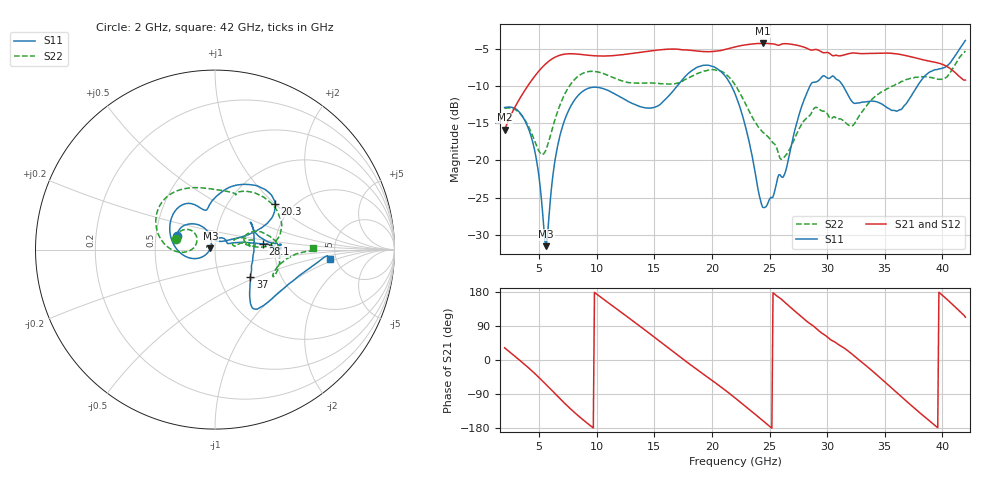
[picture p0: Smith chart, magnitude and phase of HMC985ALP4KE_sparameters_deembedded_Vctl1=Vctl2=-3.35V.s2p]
!s2p File: Measurements: S11, S21, S12, S22
# GHz S dB R 50.0
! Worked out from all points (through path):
!   401 points, 2 GHz to 42 GHz, reference 50 ohm
!   highest |S21| = -4.25 dB at 24.4 GHz (marker M1); lowest = -15.9 dB at 2 GHz (marker M2)
!   lowest |S11| = -31.5 dB at 5.6 GHz (marker M3), VSWR 1.05, Z = 47.5 + j0.726 ohm
!   |S11| at or under -10 dB: start of sweep to 16.97 GHz; 21.7 GHz to 28.5 GHz (6.799 GHz wide, 27.1 % of centre); 31.39 GHz to 37.83 GHz (6.435 GHz wide, 18.6 % of centre)
!   |S22| runs from -19.8 to -5.3 dB; largest |S21 - S12| = 0.00072
!   S11 on the Smith chart (normalised r, x): 2 GHz: 0.64, +0.11; 20.3 GHz: 1.62, +1.01; 28.1 GHz: 1.72, +0.12; 37 GHz: 1.41, -0.46; 42 GHz: 4.44, -0.78
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2  -12.89 160.0  -15.88 32.2  -15.88 32.2  -13.00 164.7
4.2  -16.28 120.6  -9.54 -24.1  -9.54 -24.1  -15.85 140.6
5.6  -31.54 163.2  -6.96 -64.7  -6.96 -64.7  -18.53 174.7
6.8  -16.69 -161.1  -5.84 -101.8  -5.84 -101.8  -12.56 -179.3
8.7  -10.80 150.2  -5.75 -155.1  -5.75 -155.1  -8.35 148.0
10.5  -10.30 123.6  -5.95 162.3  -5.95 162.3  -8.27 120.3
12.6  -11.96 110.7  -5.70 115.2  -5.70 115.2  -9.46 91.4
15.4  -12.58 99.7  -5.13 51.0  -5.13 51.0  -9.64 70.0
17.7  -8.67 74.0  -5.12 -2.5  -5.12 -2.5  -9.09 66.9
20.3  -7.51 37.4  -5.30 -60.4  -5.30 -60.4  -7.83 30.0
22  -11.01 25.0  -4.73 -100.0  -4.73 -100.0  -9.80 6.1
24.4  -26.31 70.0  -4.25 -159.7  -4.25 -159.7  -16.18 13.2
26.1  -22.28 28.2  -4.32 158.5  -4.32 158.5  -19.81 19.4
28.1  -11.45 6.9  -4.81 105.4  -4.82 105.4  -14.48 18.0
28.7  -9.53 1.0  -5.15 92.0  -5.15 92.0  -13.40 14.6
30.6  -8.73 3.6  -5.91 48.7  -5.90 48.6  -14.11 9.7
32.4  -12.33 25.5  -5.55 9.3  -5.55 9.2  -14.98 23.2
33.9  -12.01 36.6  -5.59 -28.3  -5.59 -28.4  -11.75 23.3
35.4  -13.05 10.9  -5.57 -68.5  -5.56 -68.5  -10.23 14.6
37  -12.05 -37.7  -5.95 -111.8  -5.95 -111.8  -9.07 3.0
39.5  -7.78 -52.2  -6.83 -176.1  -6.83 -176.2  -9.00 -24.4
42  -3.85 -4.6  -9.18 113.0  -9.18 113.0  -5.28 1.2
